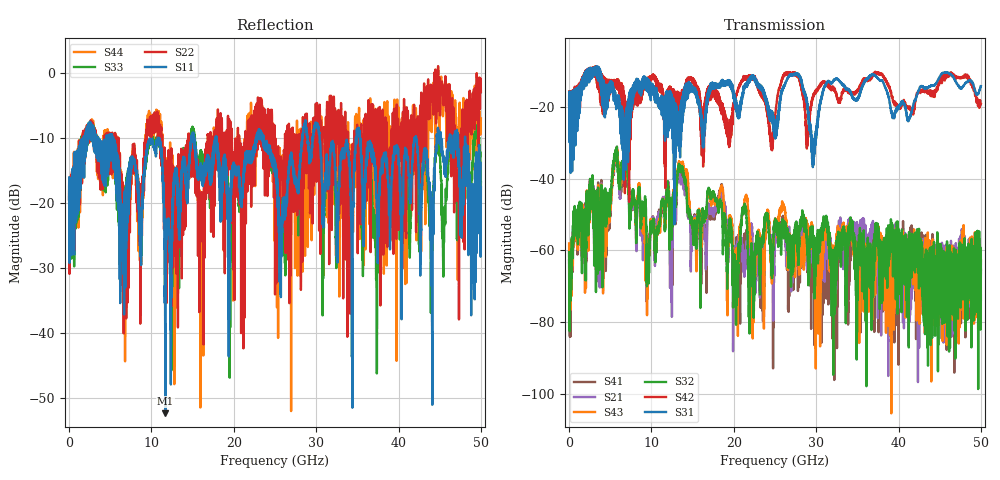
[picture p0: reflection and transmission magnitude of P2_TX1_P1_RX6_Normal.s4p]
!Keysight Technologies,N5225B,MY57041031,A.13.20.10
!Date: Friday, May 31, 2019 11:23:05
!Correction: S11(Full 4 Port(1,2,3,4))
!S12(Full 4 Port(1,2,3,4))
!S13(Full 4 Port(1,2,3,4))
!S14(Full 4 Port(1,2,3,4))
!S21(Full 4 Port(1,2,3,4))
!S22(Full 4 Port(1,2,3,4))
!S23(Full 4 Port(1,2,3,4))
!S24(Full 4 Port(1,2,3,4))
!S31(Full 4 Port(1,2,3,4))
!S32(Full 4 Port(1,2,3,4))
!S33(Full 4 Port(1,2,3,4))
!S34(Full 4 Port(1,2,3,4))
!S41(Full 4 Port(1,2,3,4))
!S42(Full 4 Port(1,2,3,4))
!S43(Full 4 Port(1,2,3,4))
!S44(Full 4 Port(1,2,3,4))
!S4P File: Measurements: <S11,S12,S13,S14>,
!<S21,S22,S23,S24>,
!<S31,S32,S33,S34>,
!<S41,S42,S43,S44>:
# Hz S  dB  R 50.0
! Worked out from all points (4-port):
!   5000 points, 10 MHz to 50 GHz, reference 50 ohm
!   strongest paths, dB at 10 MHz, 12.51 GHz, 25.01 GHz, 37.51 GHz, 50 GHz:
!     S31: -19.4, -17.3, -28.8, -12.1, -14.2
!     S42: -19.4, -15.3, -22.6, -10.4, -19.2
!     S32: -60.5, -49.1, -51.9, -55.1, -62.8
!     S43: -58.1, -48.9, -52.5, -60.1, -62.8
!     S21: -60.4, -53.3, -56.4, -60.8, -73.7
!     S41: -62.8, -55.9, -56.3, -60.1, -65.5
!   lowest |S11| = -52.3 dB at 11.69 GHz (marker M1), VSWR 1.00, Z = 49.8 - j0.121 ohm
!   |S11| at or under -10 dB: 5.36 GHz to 10.81 GHz (5.449 GHz wide, 67.4 % of centre); 17.89 GHz to 22.7 GHz (4.804 GHz wide, 23.7 % of centre); 35.31 GHz to 41.98 GHz (6.663 GHz wide, 17.2 % of centre)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
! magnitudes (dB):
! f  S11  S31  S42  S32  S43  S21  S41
! 10 MHz  -19.5  -19.4  -19.4  -60.5  -58.1  -60.4  -62.8
! 5.71 GHz  -13.1  -18.6  -13.9  -32.2  -32.3  -32.7  -33.0
! 9.47 GHz  -11.8  -14.6  -13.0  -59.5  -78.1  -62.0  -67.4
! 11.69 GHz  -52.3  -22.9  -26.4  -49.8  -49.2  -46.9  -46.7
! 21.49 GHz  -13.4  -13.5  -12.1  -49.2  -45.0  -62.3  -56.1
! 22.41 GHz  -11.7  -12.3  -11.3  -78.8  -77.2  -62.5  -61.0
! 50 GHz  -17.6  -14.2  -19.2  -62.8  -62.8  -73.7  -65.5
